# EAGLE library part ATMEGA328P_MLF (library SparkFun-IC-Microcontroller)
Datasheet SparkFun Products () () 32-Pin Atmega328 part Commonly used on Arduino compatible boards Available in QFP and QFN packages TQFP is IC-09069 QFN is non-stock
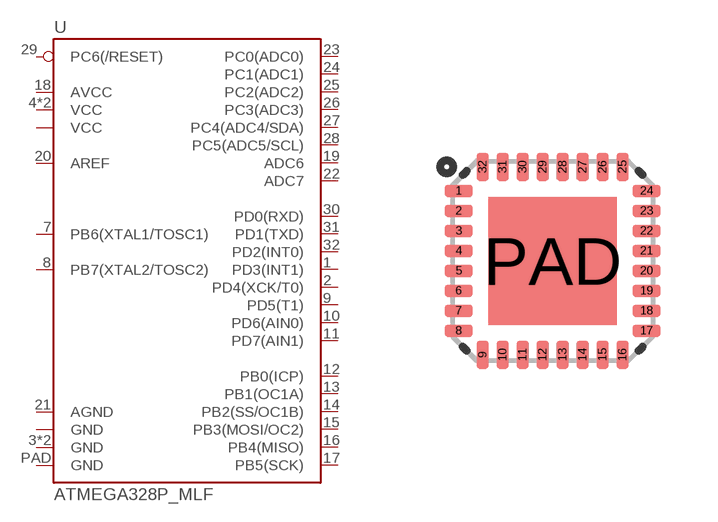
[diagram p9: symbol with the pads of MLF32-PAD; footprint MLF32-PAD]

Designator prefix U

## ATMEGA328P_MLFMLF32  [MLF32-PAD]
1  PD3(INT1)
2  PD4(XCK/T0)
3  GND
4  VCC
5  GND
6  VCC
7  PB6(XTAL1/TOSC1)
8  PB7(XTAL2/TOSC2)
9  PD5(T1)
10  PD6(AIN0)
11  PD7(AIN1)
12  PB0(ICP)
13  PB1(OC1A)
14  PB2(SS/OC1B)
15  PB3(MOSI/OC2)
16  PB4(MISO)
17  PB5(SCK)
18  AVCC
19  ADC6
20  AREF
21  AGND
22  ADC7
23  PC0(ADC0)
24  PC1(ADC1)
25  PC2(ADC2)
26  PC3(ADC3)
27  PC4(ADC4/SDA)
28  PC5(ADC5/SCL)
29  PC6(/RESET)
30  PD0(RXD)
31  PD1(TXD)
32  PD2(INT0)
PAD  GND

## Footprint MLF32-PAD (pad centres in mm)
smd 0.7 x 0.3: 1 -2.35,1.75; 2 -2.35,1.25; 3 -2.35,0.75; 4 -2.35,0.25; 5 -2.35,-0.25; 6 -2.35,-0.75; 7 -2.35,-1.25; 8 -2.35,-1.75; 17 2.35,-1.75; 18 2.35,-1.25; 19 2.35,-0.75; 20 2.35,-0.25; 21 2.35,0.25; 22 2.35,0.75; 23 2.35,1.25; 24 2.35,1.75
smd 0.3 x 0.7: 9 -1.75,-2.35; 10 -1.25,-2.35; 11 -0.75,-2.35; 12 -0.25,-2.35; 13 0.25,-2.35; 14 0.75,-2.35; 15 1.25,-2.35; 16 1.75,-2.35; 25 1.75,2.35; 26 1.25,2.35; 27 0.75,2.35; 28 0.25,2.35; 29 -0.25,2.35; 30 -0.75,2.35; 31 -1.25,2.35; 32 -1.75,2.35
smd 3.2 x 3.2: PAD 0,0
